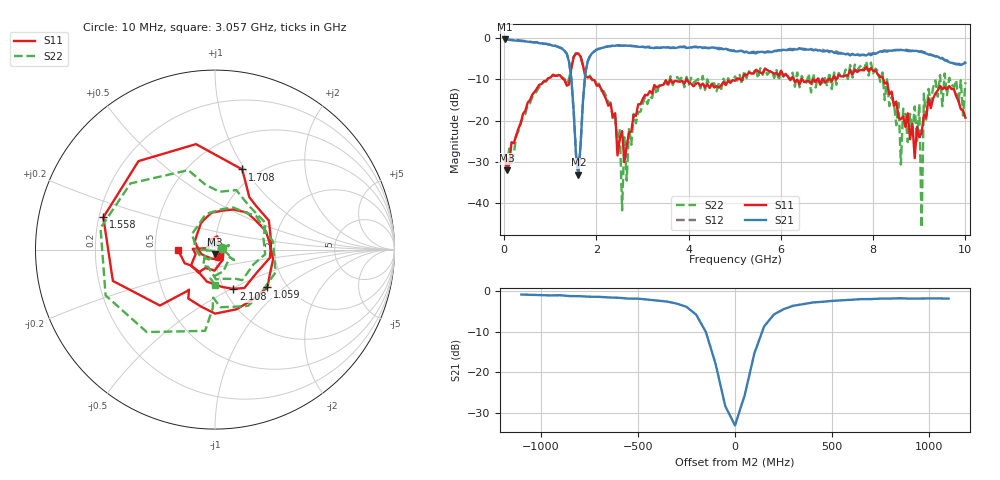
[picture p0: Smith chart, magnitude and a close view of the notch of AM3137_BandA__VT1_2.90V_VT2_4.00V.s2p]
! Date/Time: Tue, Nov 13, 2018 4:48 PM
! Network Analyzer: Agilent Technologies E8364B Rev: A.07.50.67
! Sweep from 0.010 to 10.000 GHz, 201 Points, Sweep Type: LIN
! Power Supply: 2.901 V, -0.002 A
# Hz S DB R 50
!freq MagS11 AngS11 MagS21 AngS21 MagS12 AngS12 MagS22 AngS22
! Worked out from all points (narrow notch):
!   201 points, 10 MHz to 10 GHz, reference 50 ohm
!   highest |S21| = -0.30 dB at 10 MHz (marker M1); lowest = -33.1 dB at 1.608 GHz (marker M2)
!   notch at M2: 30.2 dB deep, 186 MHz wide at half that depth
!   lowest |S11| = -32.0 dB at 59.95 MHz (marker M3), VSWR 1.05, Z = 49.9 - j2.52 ohm
!   |S11| at or under -10 dB: 1.908 GHz to 3.605 GHz (1.698 GHz wide, 61.6 % of centre); 3.962 GHz to 5.033 GHz (1.071 GHz wide, 23.8 % of centre); 8.22 GHz to end of sweep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
!   |S22| runs from -45.9 to -3.6 dB; largest |S21 - S12| = 0.036
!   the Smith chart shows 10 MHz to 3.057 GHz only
!   S11 on the Smith chart (normalised r, x): 10 MHz: 1.04, -0.07; 1.059 GHz: 1.60, -0.77; 1.558 GHz: 0.22, +0.13; 1.708 GHz: 0.85, +0.97; 2.108 GHz: 1.10, -0.51; 3.057 GHz: 0.66, -0.00
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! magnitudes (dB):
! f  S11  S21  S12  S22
! 10 MHz  -28.3  -0.3  -0.2  -27.9
! 59.95 MHz  -32.0  -0.4  -0.3  -31.0
! 1.059 GHz  -8.9  -1.8  -1.8  -8.9
! 1.409 GHz  -11.2  -5.8  -5.7  -9.7
! 1.558 GHz  -3.8  -28.3  -28.2  -3.6
! 1.608 GHz  -3.7  -33.1  -33.1  -3.8
! 1.708 GHz  -6.5  -15.3  -15.3  -6.6
! 2.108 GHz  -12.4  -2.4  -2.3  -12.8
! 2.508 GHz  -24.2  -1.8  -1.7  -22.0
! 2.557 GHz  -22.5  -1.8  -1.7  -41.7
! 2.607 GHz  -30.0  -1.8  -1.8  -24.0
! 3.057 GHz  -13.7  -2.2  -2.2  -14.2
! 3.357 GHz  -11.6  -2.4  -2.4  -11.5
! 5.005 GHz  -10.3  -3.2  -3.0  -9.3
! 6.703 GHz  -9.9  -3.0  -2.9  -8.6
! 8.352 GHz  -13.6  -3.0  -2.9  -16.5
! 8.551 GHz  -19.3  -2.9  -2.9  -15.7
! 8.601 GHz  -19.6  -2.8  -2.8  -30.6
! 9.001 GHz  -24.0  -3.3  -3.2  -16.0
! 9.051 GHz  -23.0  -3.4  -3.1  -45.9
! 9.101 GHz  -18.5  -3.6  -3.3  -13.4
! 10 GHz  -19.2  -5.9  -5.9  -10.7
